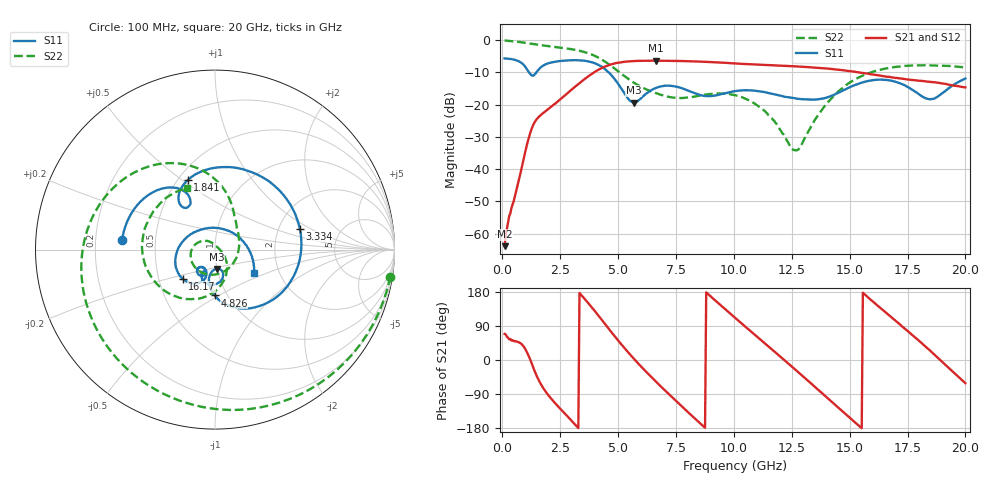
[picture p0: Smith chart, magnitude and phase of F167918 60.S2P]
!  2-Port S-parameters saved by WinCal
! VAR MeasName=S-Parameters (CALIBRATED_DATA) read from VNA (N5242A)
! VAR MeasDate=2016-11-22 10:27:47
! VAR NAME=F167918 60
! VAR FILENAME=F167918 60.S2P
! VAR DATE=2016-11-22 10:27:47
! VAR PHYS_PORTS=1,2
# Hz S DB R 50
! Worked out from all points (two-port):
!   401 points, 100 MHz to 20 GHz, reference 50 ohm
!   highest |S21| = -6.38 dB at 6.617 GHz (marker M1); lowest = -63.9 dB at 100 MHz (marker M2)
!   |S21| within 3 dB of the highest: 4.106 GHz to 14.76 GHz (10.65 GHz wide, 113 % of centre)
!   lowest |S11| = -19.3 dB at 5.672 GHz (marker M3), VSWR 1.24, Z = 49.8 - j10.8 ohm
!   |S11| at or under -10 dB: 1.152 GHz to 1.472 GHz (320.7 MHz wide, 24.4 % of centre); 4.596 GHz to end of sweep
!   |S22| runs from -34.2 to -0.1 dB; largest |S21 - S12| = 0.0031
!   S11 on the Smith chart (normalised r, x): 100 MHz: 0.32, +0.05; 1.841 GHz: 0.56, +0.53; 3.334 GHz: 2.61, +0.80; 4.826 GHz: 0.87, -0.48; 16.17 GHz: 0.66, -0.23; 20 GHz: 1.49, -0.41
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1e8  -5.68 174.1  -63.91 68.8  -62.86 76.1  -0.10 -8.8
8.96e8  -7.47 125.0  -37.65 37.6  -37.67 37.8  -0.73 -70.7
1.34375e9  -11.02 124.6  -26.15 -21.0  -26.16 -20.8  -1.22 -100.5
1.84125e9  -7.60 111.3  -22.19 -80.7  -22.19 -80.7  -1.71 -129.2
2.5875e9  -6.42 64.7  -17.85 -134.1  -17.86 -134.2  -2.38 -167.4
3.33375e9  -6.26 14.0  -13.33 176.9  -13.34 177.1  -3.30 156.3
3.43325e9  -6.30 6.8  -12.75 170.0  -12.76 170.2  -3.47 151.4
4.1795e9  -7.78 -48.6  -9.09 115.0  -9.05 115.1  -5.54 114.4
4.82625e9  -11.85 -90.4  -7.27 64.8  -7.24 64.7  -8.67 86.2
5.672e9  -19.34 -85.1  -6.48 4.0  -6.47 3.9  -13.16 60.7
6.61725e9  -14.84 -80.7  -6.38 -56.1  -6.38 -56.1  -16.39 29.7
6.7665e9  -14.51 -85.3  -6.39 -65.1  -6.38 -65.1  -16.78 22.6
8.50775e9  -16.95 -118.6  -6.66 -165.0  -6.63 -165.1  -17.22 -85.4
1.005e10  -15.82 -115.2  -7.21 111.3  -7.20 111.4  -17.09 -166.1
1.149275e10  -16.39 -130.6  -7.74 36.0  -7.70 35.8  -23.25 134.7
1.258725e10  -18.00 -129.3  -8.10 -21.8  -8.09 -21.9  -34.08 55.4
1.338325e10  -18.47 -121.6  -8.44 -64.6  -8.41 -64.5  -26.20 -25.8
1.487575e10  -15.08 -109.9  -9.51 -145.3  -9.45 -145.7  -13.82 -81.6
1.616925e10  -12.27 -137.9  -10.86 145.7  -10.85 145.7  -9.46 -128.0
1.67165e10  -12.50 -157.0  -11.40 117.5  -11.45 117.3  -8.60 -146.4
1.85075e10  -18.31 81.9  -12.94 22.9  -12.96 22.9  -7.83 158.6
2e10  -11.91 -30.7  -14.64 -61.2  -14.54 -60.8  -8.54 114.4
